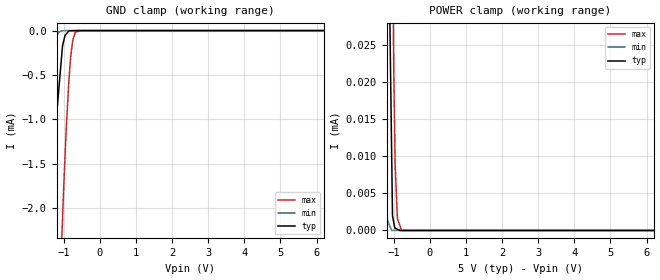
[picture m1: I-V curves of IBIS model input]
|Texas Instruments Incorporated
| Quad, Serial Input, 12-Bit, Voltage Output Digital-To-Analog Converter
| Marketing part#   Digital Voltage Range   Package-type   #pins
| DAC7714U   4.875V - 5.125V   SOIC   16
| DAC7714U/1K   4.875V - 5.125V   SOIC   16
| DAC7714U/1KG4   4.875V - 5.125V   SOIC   16
| DAC7714UB   4.875V - 5.125V   SOIC   16
| DAC7714UB/1K   4.875V - 5.125V   SOIC   16
| DAC7714UB/1KG4   4.875V - 5.125V   SOIC   16
| DAC7714UBG4   4.875V - 5.125V   SOIC   16
| DAC7714UG4   4.875V - 5.125V   SOIC   16
[IBIS Ver]   3.2
[File name]   dac7714.ibs
|SIMDE Ver   V2.2 - 201009 - Build 424
[File Rev]   1.0
[Date]   10/14/2011
[Source]
| Texas Instruments Incorporated.
| Analog-eLab Design Center, HPA
| 12500 TI Blvd
| Dallas, TX -75243
| e-mail: elab_scm_ibis@list.ti.com
[Notes]   Revision History:
| Rev 1.0: 10/14/2011
| - Initial version of the model
| - Model generated from simulations in SPECTRE
| - Model matched to SPICE simulation
| - C_comp although listed in numerical order of value are
|   obtained from varying PVT conditions. For PVT conditions for
|   each specific value refer the buffer description under
|   respective [Model]. IBIS model user is responsible for using
|   appropriate C_comp to simulate for Signal Integrity.
[Disclaimer]
| This model is designed as an aid for customers of Texas Instruments.
| TI and its licensors and suppliers make no warranties, either expressed
| or implied, with respect to this  model, including the warranties of
| merchantability or fitness for a particular purpose. The model is
| provided solely on an "as is" basis. The entire risk as to its quality
| and performance is with the customer.
[Copyright]
 (C) Copyright 2011 Texas Instruments Incorporated.All rights reserved.
|   DAC7714
[Component]   DAC7714
[Manufacturer]   TI
[Package]   |16 SOIC   -  DW package
|   typ   min   max
R_pkg   0.05587   0.02669   0.07548
L_pkg   2.73779nH   1.91487nH   3.43656nH
C_pkg   0.52613pF   0.46566pF   0.67022pF
[Pin]  signal_name   model_name   R_pin   L_pin   C_pin
1   VCC   power   0.05370   3.60200nH  0.68316pF
2   VOUTD   term   0.07527   3.22478nH  0.54751pF
3   VOUTC   term   0.05833   2.54688nH  0.46927pF
4   VREFL   term   0.03195   2.15536nH  0.51539pF
5   VREFH   term   0.03184   2.15889nH  0.51559pF
6   VOUTB   term   0.05842   2.56890nH  0.47433pF
7   VOUTA   term   0.07548   3.37714nH  0.58693pF
8   VSS   power   0.05811   3.58185nH  0.64422pF
9   GND   gnd   0.03027   3.18494nH  0.74561pF
10   SDI   input   0.06963   3.06600nH  0.54098pF
11   CLK   input   0.05344   2.41111nH  0.46566pF
12   _CS   input   0.07324   2.98171nH  0.48232pF
13   NIC   NC   0.00236   1.26007nH  0.38428pF
14   _LOADDACS   input   0.02669   1.91487nH  0.50636pF
15   _RESET   input   0.06798   3.01129nH  0.53904pF
16   RESETSEL   input   0.04813   3.43656nH  0.67022pF
[Model] term
Model_type Terminator
C_comp   1.0e-20F  1.0e-20F  1.0e-20F
|   typ   min   max
[Voltage Range]   5.0V   4.875V   5.125V
[POWER Clamp Reference]   5.0V   4.875V   5.125V
[GND Clamp Reference]   0V   0V   0V
|Ambient Temperature   25   85   -40
|Junction Temperature
[Temperature Range]   40   105   -40
| Models and submodels in the file (2): input (Input), term (Terminator)
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|   input Model
[Model]   input
Model_type   Input
Vinl = 1.575
Vinh = 3.325
|   typ   min   max
|   (nom PVT)   (fast PVT)   (slow PVT)
|C_comp from frequency sweep method (F=12.5MHz)
|Average
C_comp   1.720e-12   1.702e-12   1.721e-12
|C_comp from LC tank measurement(L=1nH)
|Average
|Resonant Frequency(Hz)   3.620e+09   3.680e+09   3.570e+09
|C_comp   1.935e-12   1.872e-12   1.990e-12
| Where nom  PVT is Nominal Process, 5V, 40C
|   Fast PVT is Strong Process,  5.125V, -40C
|   Slow PVT is Weak Process,   4.875V, 105C
[Voltage Range]   5   4.875   5.125
|Ambient Temperature   25   85   -40
|Junction Temperature
[Temperature Range]   40   105   -40
[Power Clamp Reference]   5   4.875   5.125
[GND Clamp Reference]   0   0   0
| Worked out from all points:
|   GND clamp passes 1 mA (typ) near -1.21 V on its own axis
[GND Clamp]
|   Voltage   I(typ)   I(min)   I(max)
-5V       -63.28mA   -45.87mA   -77.46mA
-1.771V   -6.453mA   -2.613mA   -13.32mA
-1.53V    -3.613mA   -1.076mA   -9.393mA
-1.246V   -1.178mA   -102.5uA   -4.778mA
-1.074V   -363.8uA   -7.289uA   -2.564mA
-1.037V   -185.6uA   -1.485uA   -2.155mA
-930.7mV  -38.31uA   -26.23nA   -1.113mA
-859mV    -5.245uA   -24.2nA    -577.7uA
-802.6mV  -1.741uA   -22.61nA   -277.1uA
-751.4mV  -1.29uA    -21.16nA   -109.7uA
-679.6mV  -657.6nA   -19.13nA   -18.16uA
10V       0A         0A         0A
[POWER Clamp]
|   Voltage   I(typ)   I(min)   I(max)
-5V       22.84mA    15.82mA    36.84mA
-1.587V   636.1uA    239.2uA    1.628mA
-1.25V    80.09uA    8.832uA    399uA
-1.173V   52.18uA    1.327uA    227.9uA
-1.105V   27.44uA    559nA      116.1uA
-1.056V   9.693uA    0A         61.49uA
-1.035V   2.022uA    0A         42.83uA
-1.002V   1.166uA    0A         23.03uA
-961.5mV  292.7nA    0A         9.003uA
-900mV    165.5nA    0A         1.706uA
-782.1mV  0A         0A         0A
10V       0A         0A         0A
